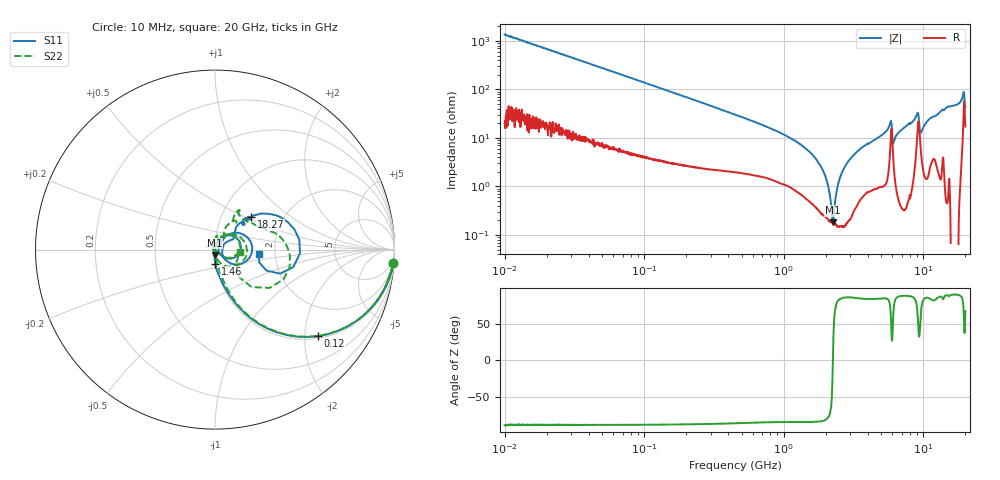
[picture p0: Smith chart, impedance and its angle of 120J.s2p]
!Keysight Technologies,P5008B,MY61100088,A.16.20.02
!Date: Monday, November 06, 2023 16:24:39
!Correction: S11(C  2-Port  )
!S21(C  2-Port  )
!S12(C  2-Port  )
!S22(C  2-Port  )
!S2P File: Measurements: S11, S21, S12, S22:Log Frequency Sweep
# Hz S  dB  R 50
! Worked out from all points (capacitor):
!   1601 points, 10 MHz to 20 GHz, reference 50 ohm
!   read as one part in series: C = 11.7 pF near 10.39 MHz
!   lowest |Z| = 182 mohm at 2.249 GHz (marker M1)
!   series resonance near 2.248 GHz, so ESL is about 430 pH
!   S11 on the Smith chart (normalised r, x): 10 MHz: 1, -27; 120 MHz: 1.06, -2.32; 1.46 GHz: 0.99, -0.16; 18.27 GHz: 1.38, +0.54; 20 GHz: 1.65, -0.09
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1e7  -0.03 -4.2  -22.70 84.9  -22.70 85.0  -0.03 -4.2
3.555162e7  -0.33 -14.4  -12.13 74.1  -12.14 74.2  -0.33 -14.4
1.199566e8  -2.53 -40.2  -3.83 48.0  -3.83 48.0  -2.57 -40.3
1.263918e8  -2.73 -41.6  -3.58 46.6  -3.58 46.6  -2.77 -41.7
4.472136e8  -10.52 -70.5  -0.56 16.3  -0.56 16.3  -10.96 -70.0
1.459613e9  -22.01 -89.3  -0.11 2.5  -0.11 2.4  -23.76 -84.2
1.589917e9  -23.32 -90.9  -0.09 1.7  -0.10 1.7  -25.03 -85.9
2.248971e9  -30.61 -94.5  -0.06 -1.6  -0.06 -1.6  -31.21 -99.0
2.89288e9  -40.31 -164.0  -0.08 -4.2  -0.09 -4.2  -38.46 -109.2
3.416178e9  -34.08 107.3  -0.11 -5.8  -0.11 -5.8  -55.12 -42.6
3.902191e9  -30.27 85.0  -0.10 -7.2  -0.10 -7.2  -36.72 48.4
4.99565e9  -28.22 73.9  -0.08 -10.7  -0.08 -10.7  -27.22 54.7
5.652411e9  -22.25 61.2  -0.21 -14.3  -0.22 -14.3  -21.29 57.8
5.899321e9  -16.70 5.9  -1.28 -13.0  -1.28 -13.0  -17.01 5.3
6.365204e9  -33.83 10.3  -0.09 -12.0  -0.09 -12.0  -35.29 83.4
6.900583e9  -28.35 40.9  -0.05 -14.5  -0.05 -14.5  -27.78 98.6
9.132954e9  -13.84 12.8  -1.49 -24.3  -1.49 -24.3  -15.12 7.0
1.013912e10  -27.61 -9.7  -0.12 -20.6  -0.12 -20.6  -45.08 57.0
1.104427e10  -22.33 33.5  -0.18 -24.9  -0.18 -24.9  -23.55 57.9
1.329228e10  -14.81 47.0  -0.25 -31.0  -0.25 -31.0  -15.38 61.5
1.827386e10  -11.32 42.1  -0.49 -50.7  -0.49 -50.7  -11.86 34.9
2e10  -12.09 -5.6  -1.65 -42.7  -1.66 -42.7  -17.16 -5.1
